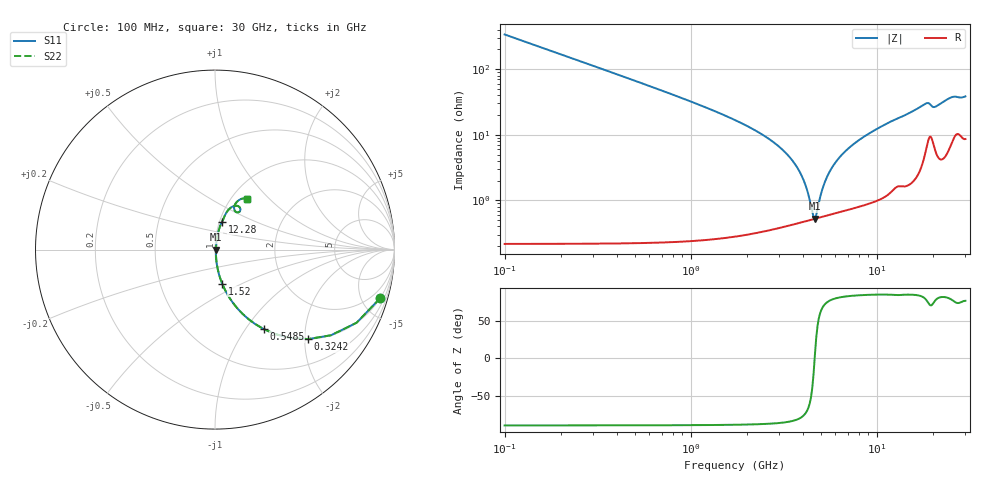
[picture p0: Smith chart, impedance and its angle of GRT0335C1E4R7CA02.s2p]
!Murata Part Number: GRT0335C1E4R7CA02
!These Parameters are Measured in Series Mode Connection
!Data Generated on Jun 19, 2026
!  o--ll--o
!Port1  Port2
!  o------o
!Operation Temp=25[degC], DC Bias Voltage=0[V]
!Freq. Start=100[MHz] Stop=30[GHz] 401[Steps]
# Hz S RI R 50
!Freq.(Hz) S11(Real) S11(Imag) S21(Real) S21(Imag) S12(Real) S12(Imag) S22(Real) S22(Imag)
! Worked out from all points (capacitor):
!   401 points, 100 MHz to 30 GHz, reference 50 ohm
!   read as one part in series: C = 4.7 pF near 249.5 MHz
!   lowest |Z| = 527 mohm at 4.66 GHz (marker M1)
!   series resonance near 4.644 GHz, so ESL is about 250 pH
!   S11 on the Smith chart (normalised r, x): 100 MHz: 1.00, -6.77; 324.2 MHz: 1.00, -2.08; 548.5 MHz: 1.00, -1.22; 1.52 GHz: 1.01, -0.40; 12.28 GHz: 1.03, +0.33; 30 GHz: 1.17, +0.75
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1e8  0.9196 -0.2716  0.0804 0.2716  0.0804 0.2716  0.9196 -0.2716
3.2425e8  0.5191 -0.4986  0.4809 0.4986  0.4809 0.4986  0.5191 -0.4986
5.485e8  0.271 -0.4426  0.729 0.4426  0.729 0.4426  0.271 -0.4426
9.2225e8  0.1121 -0.3121  0.8879 0.3121  0.8879 0.3121  0.1121 -0.3121
1.52025e9  0.0402 -0.1899  0.9598 0.1899  0.9598 0.1899  0.0402 -0.1899
2.9405e9  0.00834 -0.0676  0.9917 0.0676  0.9917 0.0676  0.00834 -0.0676
3.61325e9  0.00563 -0.0362  0.9944 0.0362  0.9944 0.0362  0.00563 -0.0362
4.06175e9  0.00507 -0.0192  0.9949 0.0192  0.9949 0.0192  0.00507 -0.0192
4.51025e9  0.0051 -0.00415  0.9949 0.00415  0.9949 0.00415  0.0051 -0.00415
4.65975e9  0.00521 0.000496  0.9948 -0.000496  0.9948 -0.000496  0.00521 0.000496
4.80925e9  0.00537 0.00499  0.9946 -0.00499  0.9946 -0.00499  0.00537 0.00499
5.10825e9  0.00578 0.0136  0.9942 -0.0136  0.9942 -0.0136  0.00578 0.0136
5.70625e9  0.00695 0.0294  0.9931 -0.0294  0.9931 -0.0294  0.00695 0.0294
6.678e9  0.00962 0.0524  0.9904 -0.0524  0.9904 -0.0524  0.00962 0.0524
8.09825e9  0.0148 0.0821  0.9852 -0.0821  0.9852 -0.0821  0.0148 0.0821
1.01165e10  0.0246 0.1199  0.9754 -0.1199  0.9754 -0.1199  0.0246 0.1199
1.228425e10  0.0397 0.1564  0.9603 -0.1564  0.9603 -0.1564  0.0397 0.1564
1.505e10  0.0594 0.1994  0.9406 -0.1994  0.9406 -0.1994  0.0594 0.1994
1.841375e10  0.1231 0.244  0.8769 -0.244  0.8769 -0.244  0.1231 0.244
2.005825e10  0.1208 0.2082  0.8792 -0.2082  0.8792 -0.2082  0.1208 0.2082
2.50665e10  0.1617 0.2849  0.8383 -0.2849  0.8383 -0.2849  0.1617 0.2849
3e10  0.1777 0.2843  0.8223 -0.2843  0.8223 -0.2843  0.1777 0.2843
